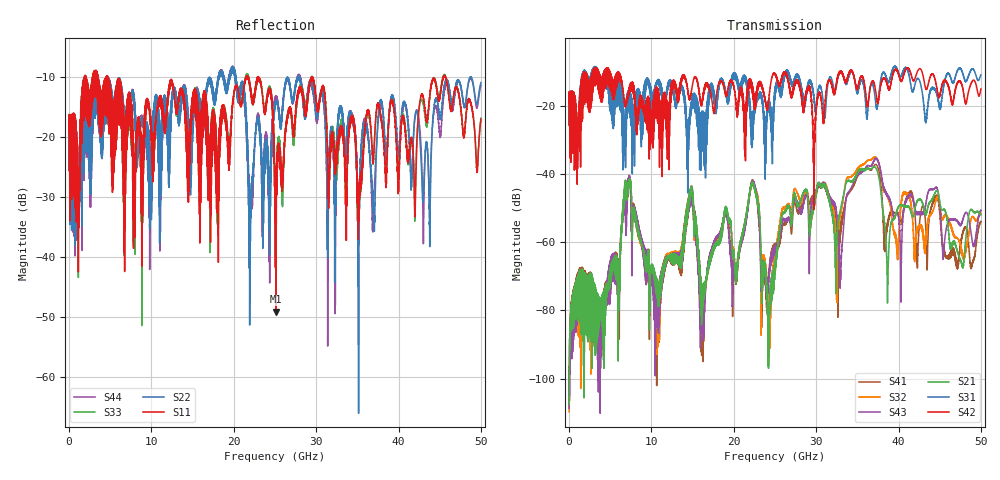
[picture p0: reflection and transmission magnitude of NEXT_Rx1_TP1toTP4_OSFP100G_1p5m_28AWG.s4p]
! Touchstone data
! Created: 27-Feb-2019 by IdEM 12 (12.1.0)
! COMMENTS
!  Created Wed Feb 27 09:43:39 2019
!  64 Port Network Data from SP1.SP block
!  freq  magS1_1  angS1_1  magS1_2  angS1_2  magS1_3  angS1_3  magS1_4  angS1_4
!  magS1_5  angS1_5  magS1_6  angS1_6  magS1_7  angS1_7  magS1_8  angS1_8
!  magS1_9  angS1_9  magS1_10  angS1_10  magS1_11  angS1_11  magS1_12  angS1_12
!  magS1_13  angS1_13  magS1_14  angS1_14  magS1_15  angS1_15  magS1_16  angS1_16
!  magS1_17  angS1_17  magS1_18  angS1_18  magS1_19  angS1_19  magS1_20  angS1_20
!  magS1_21  angS1_21  magS1_22  angS1_22  magS1_23  angS1_23  magS1_24  angS1_24
!  magS1_25  angS1_25  magS1_26  angS1_26  magS1_27  angS1_27  magS1_28  angS1_28
!  magS1_29  angS1_29  magS1_30  angS1_30  magS1_31  angS1_31  magS1_32  angS1_32
!  magS1_33  angS1_33  magS1_34  angS1_34  magS1_35  angS1_35  magS1_36  angS1_36
!  magS1_37  angS1_37  magS1_38  angS1_38  magS1_39  angS1_39  magS1_40  angS1_40
!  magS1_41  angS1_41  magS1_42  angS1_42  magS1_43  angS1_43  magS1_44  angS1_44
!  magS1_45  angS1_45  magS1_46  angS1_46  magS1_47  angS1_47  magS1_48  angS1_48
!  magS1_49  angS1_49  magS1_50  angS1_50  magS1_51  angS1_51  magS1_52  angS1_52
!  magS1_53  angS1_53  magS1_54  angS1_54  magS1_55  angS1_55  magS1_56  angS1_56
!  magS1_57  angS1_57  magS1_58  angS1_58  magS1_59  angS1_59  magS1_60  angS1_60
!  magS1_61  angS1_61  magS1_62  angS1_62  magS1_63  angS1_63  magS1_64  angS1_64
!  magS2_1  angS2_1  magS2_2  angS2_2  magS2_3  angS2_3  magS2_4  angS2_4
!  magS2_5  angS2_5  magS2_6  angS2_6  magS2_7  angS2_7  magS2_8  angS2_8
!  magS2_9  angS2_9  magS2_10  angS2_10  magS2_11  angS2_11  magS2_12  angS2_12
!  magS2_13  angS2_13  magS2_14  angS2_14  magS2_15  angS2_15  magS2_16  angS2_16
!  magS2_17  angS2_17  magS2_18  angS2_18  magS2_19  angS2_19  magS2_20  angS2_20
!  magS2_21  angS2_21  magS2_22  angS2_22  magS2_23  angS2_23  magS2_24  angS2_24
!  magS2_25  angS2_25  magS2_26  angS2_26  magS2_27  angS2_27  magS2_28  angS2_28
!  magS2_29  angS2_29  magS2_30  angS2_30  magS2_31  angS2_31  magS2_32  angS2_32
!  magS2_33  angS2_33  magS2_34  angS2_34  magS2_35  angS2_35  magS2_36  angS2_36
!  magS2_37  angS2_37  magS2_38  angS2_38  magS2_39  angS2_39  magS2_40  angS2_40
!  magS2_41  angS2_41  magS2_42  angS2_42  magS2_43  angS2_43  magS2_44  angS2_44
!  magS2_45  angS2_45  magS2_46  angS2_46  magS2_47  angS2_47  magS2_48  angS2_48
!  magS2_49  angS2_49  magS2_50  angS2_50  magS2_51  angS2_51  magS2_52  angS2_52
!  magS2_53  angS2_53  magS2_54  angS2_54  magS2_55  angS2_55  magS2_56  angS2_56
!  magS2_57  angS2_57  magS2_58  angS2_58  magS2_59  angS2_59  magS2_60  angS2_60
!  magS2_61  angS2_61  magS2_62  angS2_62  magS2_63  angS2_63  magS2_64  angS2_64
!  magS3_1  angS3_1  magS3_2  angS3_2  magS3_3  angS3_3  magS3_4  angS3_4
!  magS3_5  angS3_5  magS3_6  angS3_6  magS3_7  angS3_7  magS3_8  angS3_8
!  magS3_9  angS3_9  magS3_10  angS3_10  magS3_11  angS3_11  magS3_12  angS3_12
!  magS3_13  angS3_13  magS3_14  angS3_14  magS3_15  angS3_15  magS3_16  angS3_16
!  magS3_17  angS3_17  magS3_18  angS3_18  magS3_19  angS3_19  magS3_20  angS3_20
!  magS3_21  angS3_21  magS3_22  angS3_22  magS3_23  angS3_23  magS3_24  angS3_24
!  magS3_25  angS3_25  magS3_26  angS3_26  magS3_27  angS3_27  magS3_28  angS3_28
!  magS3_29  angS3_29  magS3_30  angS3_30  magS3_31  angS3_31  magS3_32  angS3_32
!  magS3_33  angS3_33  magS3_34  angS3_34  magS3_35  angS3_35  magS3_36  angS3_36
!  magS3_37  angS3_37  magS3_38  angS3_38  magS3_39  angS3_39  magS3_40  angS3_40
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# Hz S MA R 50
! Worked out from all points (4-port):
!   5000 points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, 10 MHz to 50 GHz, reference 50 ohm
!   strongest paths, dB at 10 MHz, 12.51 GHz, 25.01 GHz, 37.51 GHz, 50 GHz:
!     S42: -19.6, -13.3, -11.0, -19.1, -15.1
!     S31: -19.6, -14.0, -15.9, -19.1, -11.0
!     S21: -107.5, -66.1, -69.4, -39.9, -52.0
!     S43: -108.8, -65.3, -63.3, -36.4, -50.6
!     S32: -109.8, -64.8, -65.9, -36.3, -51.7
!     S41: -107.1, -66.6, -62.6, -38.3, -54.0
!   lowest |S11| = -49.2 dB at 25.11 GHz (marker M1), VSWR 1.01, Z = 50.3 + j0.113 ohm
!   |S11| at or under -10 dB: 4.66 GHz to 21.51 GHz (16.85 GHz wide, 129 % of centre); 22.94 GHz to 45.47 GHz (22.53 GHz wide, 65.9 % of centre); 45.68 GHz to end of sweep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
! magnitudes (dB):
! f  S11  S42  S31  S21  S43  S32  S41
! 10 MHz  -19.2  -19.6  -19.6  -107.5  -108.8  -109.8  -107.1
! 7.29 GHz  -16.0  -16.7  -19.3  -41.8  -40.9  -41.0  -41.6
! 10.73 GHz  -15.5  -18.3  -13.6  -76.6  -77.6  -84.6  -85.4
! 14.78 GHz  -16.9  -17.0  -20.1  -44.1  -45.3  -43.9  -45.2
! 16.2 GHz  -13.9  -17.8  -25.6  -75.6  -80.0  -74.1  -85.3
! 25.11 GHz  -49.2  -11.5  -14.8  -66.6  -62.9  -63.6  -62.5
! 50 GHz  -17.1  -15.1  -11.0  -52.0  -50.6  -51.7  -54.0
